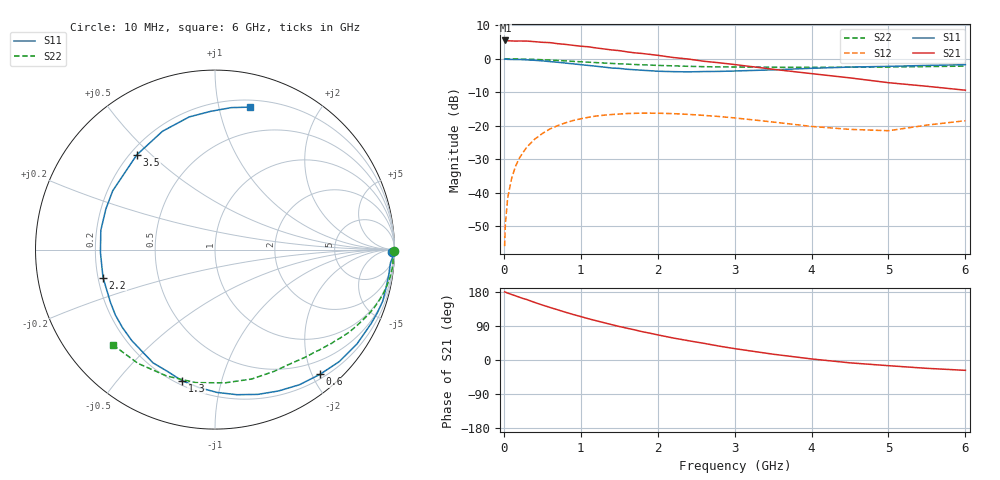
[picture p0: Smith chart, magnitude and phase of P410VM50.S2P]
! SIEMENS Small Signal Semiconductors
! BFP182
! Si NPN RF Bipolar Junction Transistor in SOT143
! VCE = 10 V  IC = 0.5 mA
! Common Emitter S-Parameters:  March  1996
# GHz  S  MA  R  50
!  f  S11  S21  S12  S22
! GHz  MAG  ANG  MAG  ANG  MAG  ANG  MAG  ANG
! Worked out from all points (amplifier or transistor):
!   36 points, 10 MHz to 6 GHz, reference 50 ohm
!   highest |S21| = 5.5 dB at 20 MHz (marker M1)
!   |S21| within 3 dB of that: start of sweep to 1.483 GHz
!   unconditionally stable (mu >= 1): 2.971 GHz to end of sweep
!   at 250 MHz: K = 0.09, MSG = 16.6 dB, |S12| = -28.0 dB
!   at 1.4 GHz: K = 0.49, MSG = 9.6 dB, |S12| = -16.6 dB
!   at 6 GHz: K = 1.22, MAG = 1.7 dB, |S12| = -18.5 dB
!   S11 on the Smith chart (normalised r, x): 10 MHz: 71, -66; 600 MHz: 0.27, -2.12; 1.3 GHz: 0.22, -0.75; 2.2 GHz: 0.22, -0.12; 3.5 GHz: 0.23, +0.45; 6 GHz: 0.26, +1.24
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0.01  0.985 -0.8  1.859 179.6  0.0016 82.9  0.9984 -0.3
0.02  0.994 -1.8  1.878 179.2  0.0034 83.6  0.9999 -0.7
0.05  0.9805 -4.3  1.859 176.5  0.0084 90.5  0.9975 -1.5
0.1  0.9782 -8.3  1.847 173.0  0.0162 83.6  0.9931 -3.0
0.15  0.9763 -12.8  1.839 169.5  0.0246 80.6  0.9951 -4.5
0.2  0.9778 -17.0  1.843 165.9  0.0327 78.8  0.9935 -6.1
0.3  0.9627 -25.3  1.838 159.5  0.0484 73.4  0.9867 -9.1
0.4  0.9498 -33.5  1.803 151.9  0.0631 68.2  0.9789 -11.9
0.6  0.9084 -49.9  1.743 138.7  0.0898 57.3  0.9561 -17.5
0.8  0.8635 -65.8  1.641 126.2  0.1106 47.7  0.9301 -22.6
1.1  0.7958 -89.2  1.511 108.9  0.1341 34.7  0.8901 -29.3
1.3  0.7527 -104.2  1.404 98.6  0.144 26.9  0.8647 -33.5
1.5  0.7192 -118.7  1.324 88.5  0.1497 20.2  0.8407 -37.2
1.8  0.6742 -139.9  1.2 74.7  0.1545 11.7  0.8138 -42.3
2.2  0.6431 -166.0  1.046 58.1  0.152 1.3  0.7854 -49.3
2.8  0.6488 159.6  0.872 36.6  0.1376 -9.7  0.7567 -59.9
3.5  0.6844 129.6  0.698 15.3  0.1139 -16.0  0.7495 -74.2
4  0.7215 113.9  0.601 2.8  0.098 -13.2  0.7445 -85.7
4.5  0.7531 101.0  0.519 -7.5  0.0885 -7.1  0.7488 -98.2
5  0.771 91.7  0.44 -15.0  0.0845 6.3  0.754 -110.9
5.5  0.7964 83.4  0.389 -22.0  0.1025 13.4  0.7656 -124.1
6  0.8173 76.2  0.34 -27.3  0.1192 15.1  0.7777 -136.9
